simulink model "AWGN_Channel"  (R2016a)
settings: Solver=ode3  StartTime=0.0  StopTime=6  FixedStep=1/5000000  RelTol=1e-3
libraries: commchan3 x1

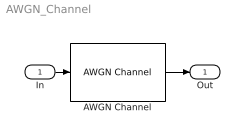
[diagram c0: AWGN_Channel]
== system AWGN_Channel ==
  In : Inport
  AWGN Channel : commchan3/AWGN Channel  InputProcessing=Columns as channels (frame based)  seed=67  noiseMode="Signal to noise ratio  (Eb/No)"  EbNodB=10  EsNodB=10  SNRdB=10  bitsPerSym=2  Ps=1  Tsym=1/5000000  variance=1
  Out : Outport
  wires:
  In/1 -> AWGN Channel/1
  AWGN Channel/1 -> Out/1
